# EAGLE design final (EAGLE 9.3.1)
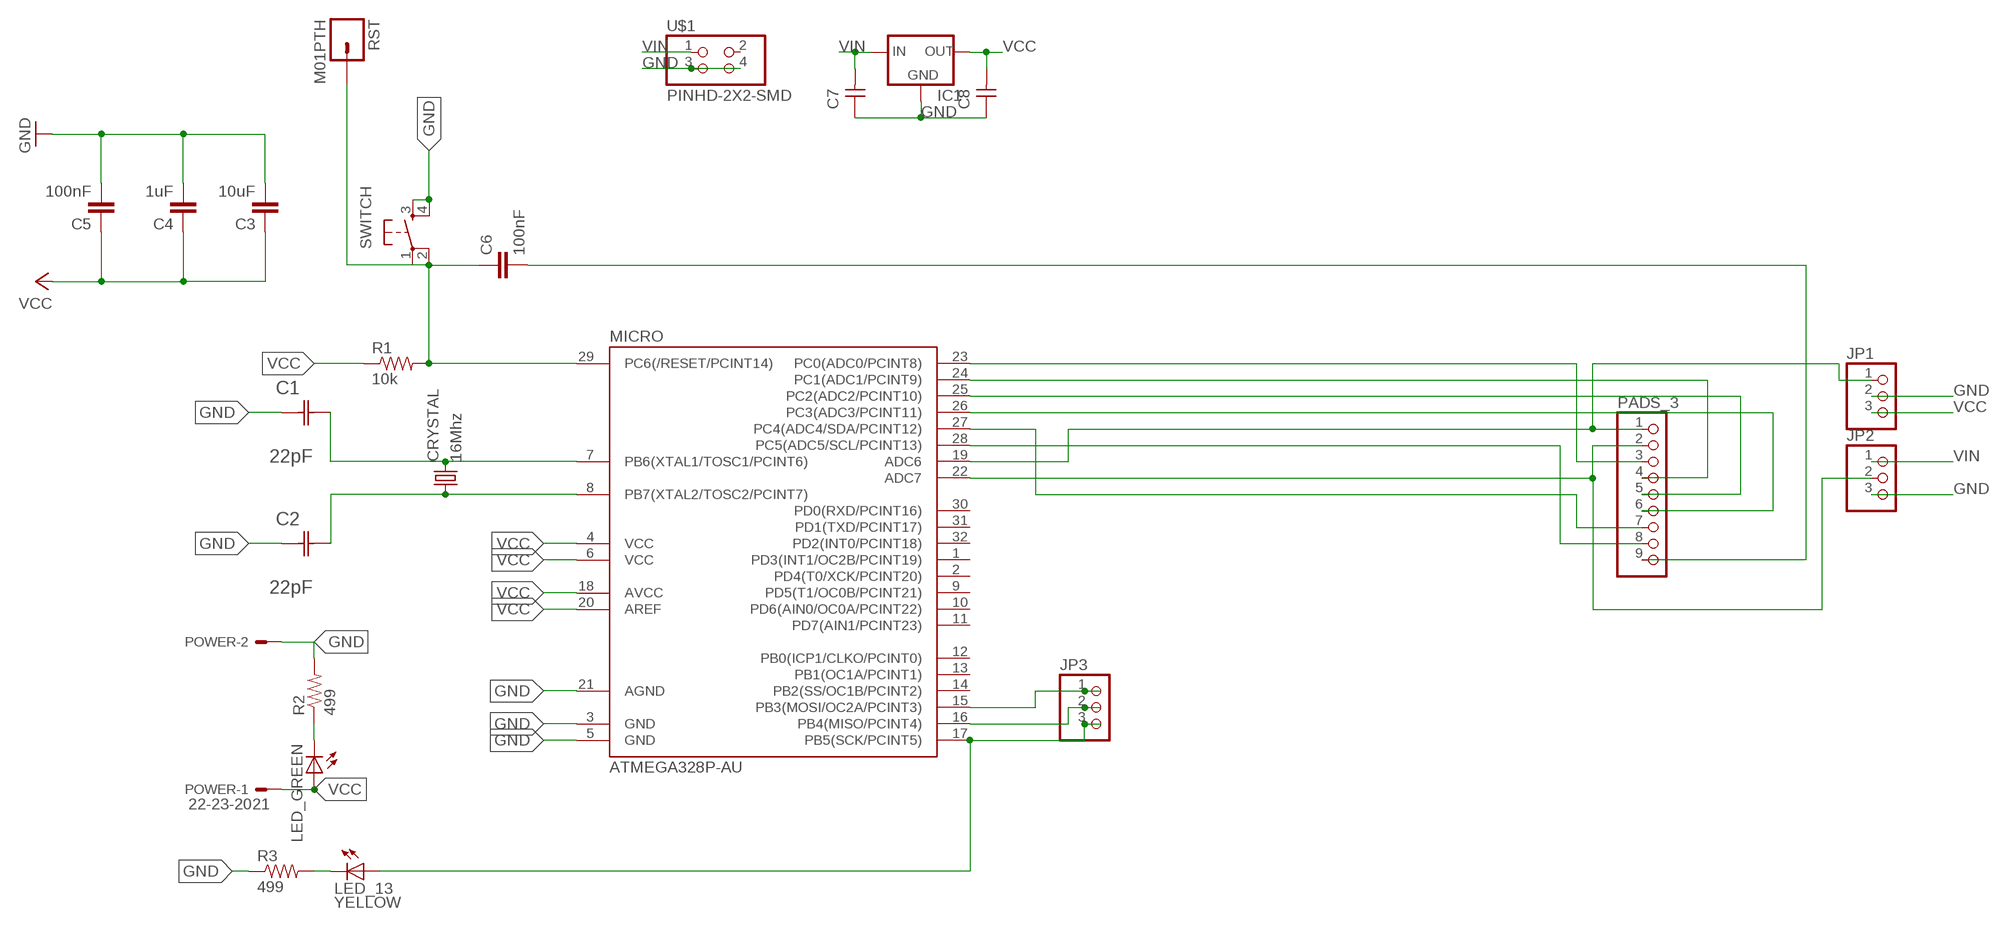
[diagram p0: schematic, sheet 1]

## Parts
C1  22pF  0612ZC225MAT2A  [CAPC3216X178N]
C2  22pF  0612ZC225MAT2A  [CAPC3216X178N]
C3  10uF  CAP1206  [1206]
C4  1uF  CAP1206  [1206]
C5  100nF  CAP1206  [1206]
C6  100nF  CAP1206  [1206]
C7  CAP-UNPOLARIZED  [C1206]
C8  CAP-UNPOLARIZED  [C1206]
CRYSTAL  16Mhz  CSM-7X-DU  [CSM-7X-DU]
IC1  78XXL  [78XXL]
JP1  PINHD-1X3  [1X03]
JP2  PINHD-1X3  [1X03]
JP3  PINHD-1X3  [1X03]
LED_13  YELLOW  LED1206  [1206]
LED_GREEN  LED1206  [1206]
MICRO  ATMEGA328P-AU  ATMEGA48/88/168-AU  [TQFP32-08]
PADS_3  PINHD-1X9  [1X09]
POWER  22-23-2021  [22-23-2021]
R1  10k  RESISTOR1206  [1206]
R2  499  RESISTOR1206  [1206]
R3  499  RESISTOR1206  [1206]
RST  M01PTH  [1X01]
SWITCH  6MM_SWITCH6MM_SWITCH  [6MM_SWITCH]
U$1  PINHD-2X2-SMD  [2X02SMD]

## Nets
GND: C1.1(C1) C2.1(C1) C3.2 C4.2 C5.2 C7.1 C8.1 IC1.GND JP1.2 JP2.3 MICRO.3(GND) MICRO.5(GND) MICRO.21(AGND) POWER.2 R2.2 R3.1 SWITCH.3(S) SWITCH.4(S1) U$1.3 U$1.4
N$1: JP3.3 LED_13.1(A) MICRO.17(PB5(SCK/PCINT5))
N$2: C1.2(C2) CRYSTAL.2 MICRO.7(PB6(XTAL1/TOSC1/PCINT6))
N$3: C6.2 PADS_3.9
N$4: JP3.1 MICRO.15(PB3(MOSI/OC2A/PCINT3))
N$5: JP3.2 MICRO.16(PB4(MISO/PCINT4))
N$9: C2.2(C2) CRYSTAL.1 MICRO.8(PB7(XTAL2/TOSC2/PCINT7))
N$13: JP1.1 MICRO.19(ADC6) PADS_3.1
N$14: JP2.2 MICRO.22(ADC7) PADS_3.2
N$15: MICRO.23(PC0(ADC0/PCINT8)) PADS_3.3
N$16: MICRO.24(PC1(ADC1/PCINT9)) PADS_3.4
N$17: MICRO.25(PC2(ADC2/PCINT10)) PADS_3.5
N$18: MICRO.26(PC3(ADC3/PCINT11)) PADS_3.6
N$19: MICRO.27(PC4(ADC4/SDA/PCINT12)) PADS_3.7
N$25: MICRO.28(PC5(ADC5/SCL/PCINT13)) PADS_3.8
N$26: LED_GREEN.2(C) R2.1
N$27: LED_13.2(C) R3.2
N$28: C6.1 MICRO.29(PC6(/RESET/PCINT14)) R1.2 RST.1 SWITCH.1(P) SWITCH.2(P1)
VCC: C3.1 C4.1 C5.1 C8.2 IC1.OUT JP1.3 LED_GREEN.1(A) MICRO.4(VCC) MICRO.6(VCC) MICRO.18(AVCC) MICRO.20(AREF) POWER.1 R1.1
VIN: C7.2 IC1.IN JP2.1 U$1.1
Unconnected: MICRO.1(PD3(INT1/OC2B/PCINT19)) MICRO.2(PD4(T0/XCK/PCINT20)) MICRO.9(PD5(T1/OC0B/PCINT21)) MICRO.10(PD6(AIN0/OC0A/PCINT22)) MICRO.11(PD7(AIN1/PCINT23)) MICRO.12(PB0(ICP1/CLKO/PCINT0)) MICRO.13(PB1(OC1A/PCINT1)) MICRO.14(PB2(SS/OC1B/PCINT2)) MICRO.30(PD0(RXD/PCINT16)) MICRO.31(PD1(TXD/PCINT17)) MICRO.32(PD2(INT0/PCINT18)) U$1.2

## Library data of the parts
C1 C2 = AVX_By_element14_Batch_1:0612ZC225MAT2A: Capacitor 1206; MPN: 0612ZC225MAT2A; OC_FARNELL: -; OC_NEWARK: 12N3209; SUPPLIER: AVX; TOLERANCE: ±20%; VALUE: 2.2µF; VOLTAGERATING: 10V
C3-C6 = 01_SparkFun:CAP: Capacitor
C7 C8 = fab:CAP-UNPOLARIZED
CRYSTAL = 01_FAB_Hello:CSM-7X-DU: SMD CRYSTAL; OC_FARNELL: unknown; OC_NEWARK: unknown
IC1 = v-reg:78XXL: VOLTAGE REGULATOR
JP1-JP3 = pinhead:PINHD-1X3: PIN HEADER
LED_13 LED_GREEN = 01_FAB_Hello:LED
MICRO = atmega8:ATMEGA48/88/168
PADS_3 = pinhead:PINHD-1X9: PIN HEADER
POWER = con-molex:22-23-2021: .100" (2.54mm) Center Header - 2 Pin; MF: MOLEX; MPN: 22-23-2021; OC_FARNELL: 1462926; OC_NEWARK: 25C3832
R1-R3 = 01_SparkFun:RESISTOR: Resistor
RST = 01_SparkFun:M01: Header 1
SWITCH = 01_FAB_Hello:6MM_SWITCH: OMRON SWITCH
U$1 = fab:PINHD-2X2-SMD

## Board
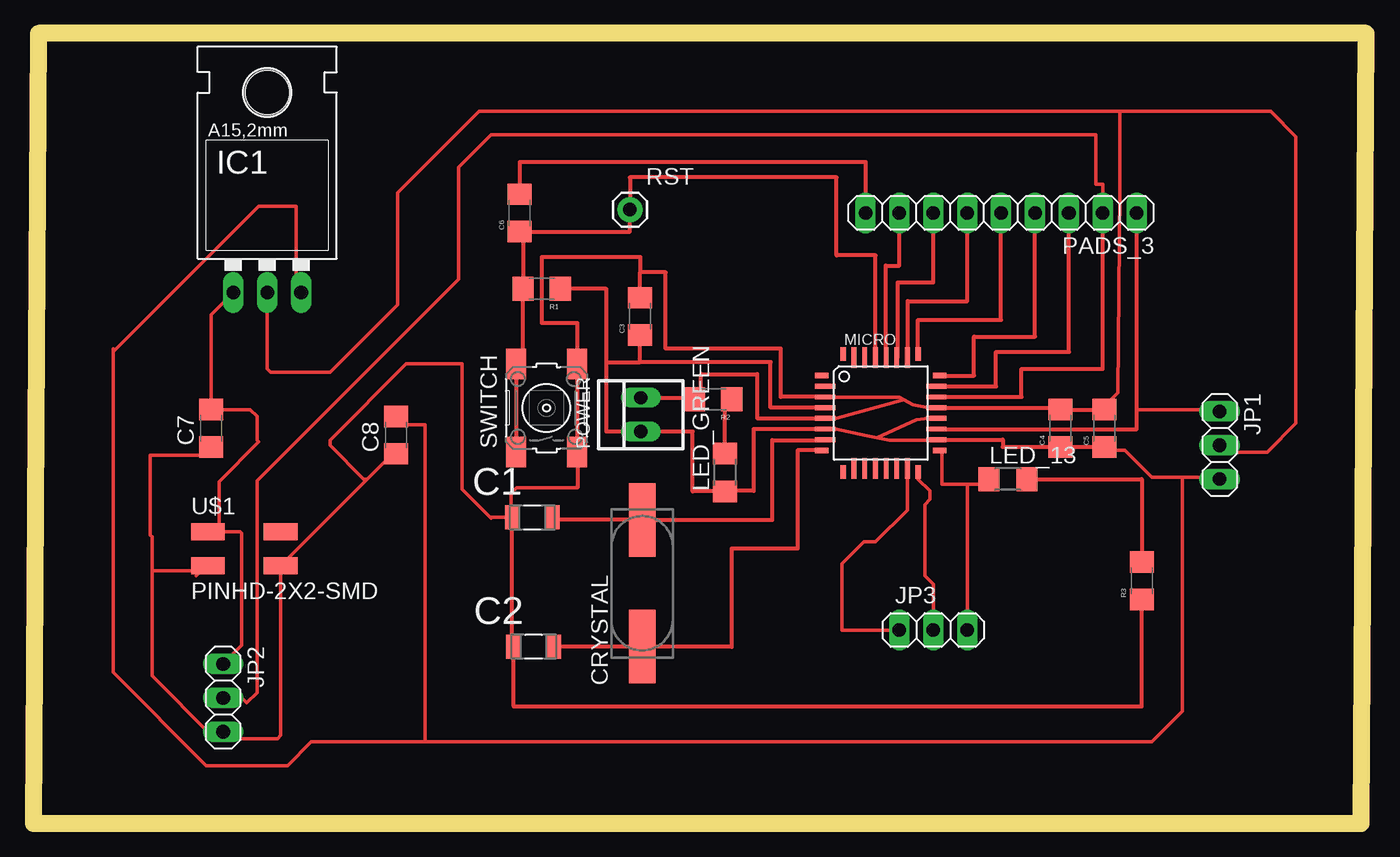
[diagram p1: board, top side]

Size 99.87 x 59.17 mm. Coordinates in mm from the lower left corner, seen from the top.
Outline: 0,0 99.49,0 99.87,59.17 0.38,59.17 0,0
Copper layers (1*16): Top 0.035mm / dielectric 1.5mm / Bottom 0.035mm
Design rules "default *": minimum track width 10mil, minimum drill 24mil, track to track 10mil, track to pad 8mil, pad to pad 8mil, via to via 8mil, smd to smd 8mil, copper to edge 40mil, drill to drill 8mil, minimum pad ring 10mil, minimum via ring 8mil, stop-mask expansion 4mil, vias tented up to drill 0mil, thermal gap 10mil

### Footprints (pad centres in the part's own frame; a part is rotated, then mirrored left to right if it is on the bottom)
CAPC3216X178N = smd 1.118 x 1.803: 1 -1.499,0; 2 1.499,0
1206 = smd 1.6 x 1.8: 1 -1.4,0; 2 1.4,0
C1206 = smd 1.6 x 1.8: 1 -1.4,0; 2 1.4,0
CSM-7X-DU = smd 5.5 x 2: 1 -4.75,0; 2 4.75,0
78XXL = drill 1.016 long: GND 0,-3.81; IN -2.54,-3.81; OUT 2.54,-3.81 | hole 3.302: 0,11.176
1X03 = drill 1.016 long: 1 -2.54,0; 2 0,0; 3 2.54,0
1206' = smd 1.6 x 1.803: 1 -1.422,0; 2 1.422,0
TQFP32-08 = smd 1.016 x 0.406: 1 -4.42,2.8; 8 -4.42,-2.8; 17 4.42,-2.8; 24 4.42,2.8 | smd 1.524 x 0.356: 2 -4.166,2; 3 -4.166,1.2; 4 -4.166,0.4; 5 -4.166,-0.4; 6 -4.166,-1.2; 7 -4.166,-2; 18 4.166,-2; 19 4.166,-1.2; 20 4.166,-0.4; 21 4.166,0.4; 22 4.166,1.2; 23 4.166,2 | smd 0.406 x 1.016: 9 -2.8,-4.42; 16 2.8,-4.42; 25 2.8,4.42; 32 -2.8,4.42 | smd 0.356 x 1.524: 10 -2,-4.166; 11 -1.2,-4.166; 12 -0.4,-4.166; 13 0.4,-4.166; 14 1.2,-4.166; 15 2,-4.166; 26 2,4.166; 27 1.2,4.166; 28 0.4,4.166; 29 -0.4,4.166; 30 -1.2,4.166; 31 -2,4.166
1X09 = drill 1.016 long: 1 -10.16,0; 2 -7.62,0; 3 -5.08,0; 4 -2.54,0; 5 0,0; 6 2.54,0; 7 5.08,0; 8 7.62,0; 9 10.16,0
22-23-2021 = drill 1 long: 1 -1.27,0; 2 1.27,0
1X01 = drill 1.016 pad 1.88: 1 0,0
6MM_SWITCH = smd 2.286 x 1.524: 1 -3.302,2.286; 2 3.302,2.286; 3 -3.302,-2.286; 4 3.302,-2.286
2X02SMD = smd 2.54 x 1.27: 1 -2.54,1.27; 2 2.92,1.27; 3 -2.54,-1.27; 4 2.92,-1.27

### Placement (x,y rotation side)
C1  37.39,22.91 0 top
C2  37.49,13.23 0 top
C3  45.47,37.97 90 top
C4  76.96,29.59 90 top
C5  80.26,29.59 90 top
C6  36.45,45.72 90 top
C7  13.34,29.59 90 top
C8  27.18,29.08 90 top
CRYSTAL  45.62,17.98 90 top
IC1  17.53,43.56 0 top
JP1  88.9,28.32 270 top
JP2  14.22,9.4 270 top
JP3  67.44,14.48 0 top
LED_13  YELLOW  [1206']  73.03,25.78 0 top
LED_GREEN  [1206']  51.82,26.29 90 top
MICRO  63.5,30.73 0 top
PADS_3  72.52,45.72 180 top
POWER  45.52,30.61 90 top
R1  38.1,40.03 180 top
R2  50.93,31.75 180 top
R3  83.06,18.16 90 top
RST  44.7,45.97 0 top
SWITCH  38.46,31.12 90 top
U$1  15.62,20.57 0 top

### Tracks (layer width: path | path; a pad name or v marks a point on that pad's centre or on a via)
GND
  Top 0.254: MICRO.3 59.36,31.91 64.89,31.91 | 64.89,31.91 65.91,31.37 67.06,31.12 | 59.94,30.35 60.2,30.35 65.07,31.7 | 65.07,31.7 65.21,31.74 | 64.89,31.91 65.07,31.7 | 25.02,25.78 U$1.4 | 25.02,25.78 26.67,27.43 27.18,27.43 C8.1 27.18,28.19 | 13.21,27.94 C7.1 12.7,27.56 8.76,27.56 8.76,21.59 8.89,21.46 8.89,18.92 | 12.57,18.92 12.95,19.3 U$1.3 | 12.57,18.92 12.19,18.54 | 18.29,19.3 U$1.4 | 88.9,28.45 JP1.2 89.41,27.81 92.46,27.81 94.62,29.97 94.62,51.44 92.71,53.34 81.41,53.34 | C5.2 80.26,31.24 81.28,32.26 81.41,47.37 81.41,53.34 | 17.53,39.09 IC1.GND 17.53,34.04 17.78,33.78 22.23,33.78 27.3,38.86 27.3,47.24 33.4,53.34 81.41,53.34 | 40.77,25.15 36.2,25.15 35.81,24.77 35.81,22.99 C1.1 34.34,22.91 34.29,22.86 32.13,25.02 32.13,34.42 27.94,34.42 22.23,28.7 22.23,28.32 24.77,25.78 25.02,25.78 | U$1.4 18.54,6.6 18.29,6.35 14.73,6.35 14.48,6.6 | 14.48,6.6 JP2.3 | 14.48,6.6 13.34,6.6 8.89,11.05 8.89,18.92 | 8.89,18.92 12.57,18.92
  Top 0.305: MICRO.5 | MICRO.21 | C1.1 35.89,13.23 C2.1 35.99,8.76 83.06,8.76 R3.1 | C1.1 35.81,22.91 | MICRO.5 59.33,30.35 54.23,30.35 54.23,33.66 50.04,33.66 50.04,31.62 50.03,31.62 R2.2 50.03,31.88 POWER.2 | C1.1 35.94,22.91 | MICRO.21 76.96,31.13 C4.2 C5.2 | 59.94,30.35 MICRO.5 | MICRO.21 67.06,31.12 | MICRO.3 56.01,31.93 56.01,35.56 47.37,35.56 47.37,41.27 45.47,41.27 | C3.2 45.47,41.27 | SWITCH.3 40.77,27.81 | 40.77,27.81 40.77,25.15 | 40.77,27.81 40.77,33.78 40.74,33.78 SWITCH.4 40.77,34.42 40.77,37.46 38.1,37.46 38.1,42.42 45.47,42.42 45.47,41.27
N$1
  Top 0.254: MICRO.17 68.07,27.78 68.07,25.4 69.98,25.4 | 69.98,25.4 71.22,25.4 LED_13.1 | JP3.3 69.98,25.4
N$2
  Top 0.305: 38.89,22.73 C1.2 38.89,22.73 | MICRO.7 59.33,28.7 55.37,28.7 55.37,22.73 CRYSTAL.2 38.89,22.73
N$3
  Top 0.305: PADS_3.9 62.36,49.53 36.45,49.53 C6.2
N$4
  Top 0.254: MICRO.15 65.5,23.46 63.12,21.08 62.23,21.08 60.58,19.43 60.58,14.48 JP3.1
N$5
  Top 0.254: JP3.2 67.44,17.91 66.8,18.54 66.8,23.88 67.18,24.26 67.18,24.89 66.3,25.77 MICRO.16
N$9
  Top 0.305: 38.99,13.21 C2.2 | MICRO.8 57.28,27.94 57.28,20.57 52.32,20.57 52.32,13.21 45.62,13.21 CRYSTAL.1 C2.2 | C2.2
N$13
  Top 0.254: 82.68,30.99 88.9,30.99 JP1.1
  Top 0.305: MICRO.19 82.68,29.53 82.68,30.99 PADS_3.1
N$14
  Top 0.254: 80.01,45.72 PADS_3.2 | JP2.2 15.62,9.4 16,9.02 16.76,9.78 16.76,25.65 31.88,40.77 31.88,49.15 34.29,51.56 79.63,51.56 79.63,47.88 80.14,47.88 80.14,45.59
  Top 0.305: MICRO.22 74.04,31.93 74.04,34.04 80.14,34.04 80.14,45.59 PADS_3.2
N$15
  Top 0.305: MICRO.23 72.14,32.73 72.14,35.31 77.6,35.31 PADS_3.3
N$16
  Top 0.305: MICRO.24 70.48,33.53 70.48,36.45 75.06,36.45 PADS_3.4
N$17
  Top 0.305: MICRO.25 66.29,37.72 72.52,37.72 PADS_3.5
N$18
  Top 0.305: MICRO.26 65.53,34.9 65.53,39.12 69.98,39.12 PADS_3.6
N$19
  Top 0.305: MICRO.27 64.77,34.9 64.77,40.51 67.44,40.51 PADS_3.7
N$25
  Top 0.305: MICRO.28 63.88,34.9 63.88,41.78 64.9,41.78 PADS_3.8
N$26
  Top 0.305: 52.7,31.5 R2.1 52.33,31.37 51.82,31.37 LED_GREEN.2
N$27
  Top 0.305: LED_13.2 83.06,25.78 R3.2
N$28
  Top 0.305: MICRO.29 63.12,34.9 63.12,42.55 60.2,42.55 60.2,48.39 44.7,48.39 RST.1 44.7,44.32 36.7,44.32 | R1.2 36.45,40.03 | R1.2 36.7,34.42 SWITCH.2 SWITCH.1 | C6.1 36.7,44.32 | 36.7,44.32 R1.2
VCC
  Top 0.254: 60.02,29.54 62.48,29.04 63.23,28.89 | 63.23,28.89 64.14,28.7 67.67,28.7 | MICRO.20 67.06,30.33 67.06,30.35 66.17,30.23 63.23,28.89 | 86.11,25.91 83.82,25.91 81.79,27.94 80.26,27.94 C5.1 | 86.11,25.91 88.9,25.91 JP1.3 | 27.18,29.97 C8.2 27.82,29.84 29.34,29.84 29.34,6.1 | 86.11,25.91 86.11,8.38 83.82,6.1 29.34,6.1 | 29.34,6.1 20.83,6.1 19.05,4.32 12.95,4.32 5.97,11.3 5.97,35.31 | 5.97,35.56 5.97,35.31 | 5.97,35.31 16.89,46.23 19.69,46.23 19.69,40.13 IC1.OUT
  Top 0.305: MICRO.18 | MICRO.20 67.06,30.35 | MICRO.4 55.25,31.13 55.25,34.54 45.47,34.54 | 42.93,34.54 42.93,40.03 R1.1 | 42.93,34.54 42.93,29.34 POWER.1 49.4,29.34 49.4,24.87 LED_GREEN.1 51.82,24.89 53.98,24.89 53.98,29.53 MICRO.6 60.02,29.54 | 67.67,28.7 MICRO.18 | MICRO.18 72.64,28.73 72.64,28.19 C4.1 C5.1 | 42.93,34.54 45.47,34.54 | 45.47,34.54 C3.1 45.85,36.57 45.85,36.32
VIN
  Top 0.254: IC1.IN 13.34,38.1 C7.2 | C7.2 13.46,31.24 13.97,31.24 C7.2 | 13.21,21.84 U$1.1 13.84,21.84 | C7.2 16.25,30.99 16.76,30.48 16.76,28.7 16.89,28.58 13.91,25.59 13.91,21.91 13.84,21.84 | 13.84,21.84 15.49,21.84 15.62,21.72 15.62,13.33 JP2.1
